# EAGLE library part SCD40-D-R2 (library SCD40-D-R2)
Air Quality Sensor CO2 Sensor 2.5V/3.3V/5V 20-Pin SMD EP Source: Datasheet
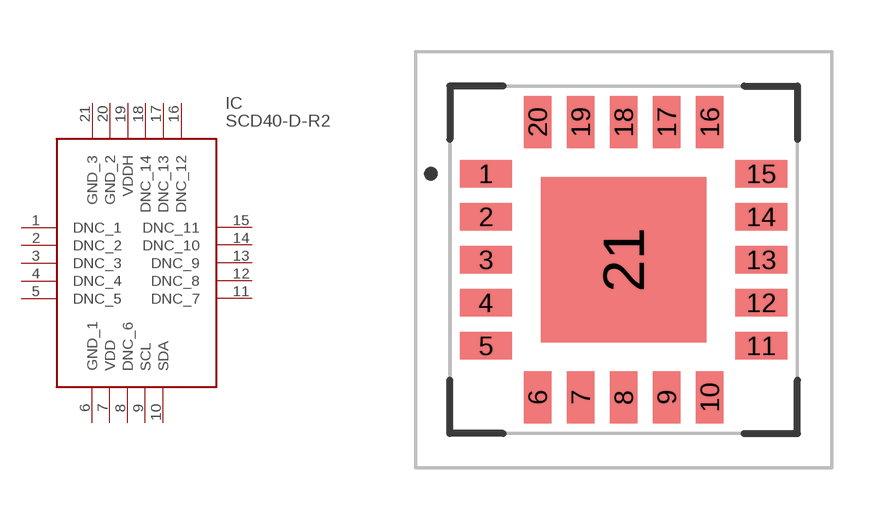
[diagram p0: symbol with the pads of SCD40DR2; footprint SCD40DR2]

Designator prefix IC

## SCD40-D-R2 (Arrow_Part_Number: SCD40-D-R2; Arrow_Price-Stock: https://www.arrow.com/en/products/scd40-d-r2/sensirion-ag?region=nac; Description: Air Quality Sensor CO2 Sensor 2.5V/3.3V/5V 20-Pin SMD EP; Height: 6.8mm; Manufacturer_Name: Sensirion; Manufacturer_Part_Number: SCD40-D-R2; Mouser_Part_Number: 403-SCD40-D-R2; Mouser_Price-Stock: https://www.mouser.co.uk/ProductDetail/Sensirion/SCD40-D-R2?qs=HBWAp0VN4RjIKW%252BlMeZn1w%3D%3D)  [SCD40DR2]
1  DNC_1
2  DNC_2
3  DNC_3
4  DNC_4
5  DNC_5
6  GND_1
7  VDD
8  DNC_6
9  SCL
10  SDA
11  DNC_7
12  DNC_8
13  DNC_9
14  DNC_10
15  DNC_11
16  DNC_12
17  DNC_13
18  DNC_14
19  VDDH
20  GND_2
21  GND_3

## Footprint SCD40DR2 (pad centres in mm)
SCD40-D-R2-1
smd 1.5 x 0.8: 1 -4,2.5; 2 -4,1.25; 3 -4,0; 4 -4,-1.25; 5 -4,-2.5; 11 4,-2.5; 12 4,-1.25; 13 4,0; 14 4,1.25; 15 4,2.5
smd 0.8 x 1.5: 6 -2.5,-4; 7 -1.25,-4; 8 0,-4; 9 1.25,-4; 10 2.5,-4; 16 2.5,4; 17 1.25,4; 18 0,4; 19 -1.25,4; 20 -2.5,4
smd 4.8 x 4.8: 21 0,0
